|Texas Instruments Incorporated
| Marketing Part # : LMKDB1XXX
| Voltage Range : 1.8-3.3V
| Package-type: QFN
| #pins/pkg drawing : 40-pin RSL
[IBIS Ver] 3.2
[File name] lmkdb1xxx.ibs
[File Rev] 1.0
[Date] 09/07/2023
[Source]
| Texas Instruments Incorporated.
| 12500 TI Blvd
| Dallas, TX -75243
[Notes] Revision History:
| Rev 1.0: 09/07/2023
| - Initial version of the model
| - Model generated from simulations in TISPICE/SPECTRE
| - C_comp although listed in numerical order of value are
| obtained from varying PVT conditions. For PVT conditions for
| each specific value refer the buffer description under
| respective [Model]. IBIS model user is responsible for using
| appropriate C_comp to simulate for Signal Integrity.
| - Warnings regarding combined Non-monotonicity of various models have been
| reviewed and considered minor and can be ignored.
[Disclaimer]
| This model is designed as an aid for customers of Texas Instruments.
| TI and its licensors and suppliers make no warranties, either expressed
| or implied, with respect to this model, including the warranties of
| merchantability or fitness for a particular purpose. The model is
| provided solely on an "as is" basis. The entire risk as to its quality
| and performance is with the customer.
| This model is subject to change without notice. Texas Instruments
| Incorporated is not responsible for updating this model.
[Copyright]
(C) Copyright 2023 Texas Instruments Incorporated. All rights reserved.
| Component LMKDB1120 (per package)
[Component] LMKDB1120
[Manufacturer] Texas Instruments Incorporated
[Package] |80 GQFN
| variable typ min max
R_pkg 0.111 0.052 0.169
L_pkg 2.02nH 1.12nH 2.9nH
C_pkg 0.163pF 0.062pF 0.264pF
| pin number (pin name) mapping to model name
[Pin] signal_name model_name R_pin L_pin C_pin
1   CLKIN_P   ck_in   NA   NA   NA
2   CLKIN_N   ck_in   NA   NA   NA
3   CLK0_P   ck_out   NA   NA   NA
4   CLK0_N   ck_out   NA   NA   NA
5   CLK1_P   ck_out   NA   NA   NA
6   CLK1_N   ck_out   NA   NA   NA
7   CLK2_P   ck_out   NA   NA   NA
8   CLK2_N   ck_out   NA   NA   NA
9   CLK3_P   ck_out   NA   NA   NA
10   CLK3_N   ck_out   NA   NA   NA
11   CLK4_P   ck_out   NA   NA   NA
12   CLK4_N   ck_out   NA   NA   NA
13   CLK5_P   ck_out   NA   NA   NA
14   CLK5_N   ck_out   NA   NA   NA
15   CLK6_P   ck_out   NA   NA   NA
16   CLK6_N   ck_out   NA   NA   NA
17   CLK7_P   ck_out   NA   NA   NA
18   CLK7_N   ck_out   NA   NA   NA
19   CLK8_P   ck_out   NA   NA   NA
20   CLK8_N   ck_out   NA   NA   NA
21   CLK9_P   ck_out   NA   NA   NA
22   CLK9_N   ck_out   NA   NA   NA
23   CLK10_P   ck_out   NA   NA   NA
24   CLK10_N   ck_out   NA   NA   NA
25   CLK11_P   ck_out   NA   NA   NA
26   CLK11_N   ck_out   NA   NA   NA
27   CLK12_P   ck_out   NA   NA   NA
28   CLK12_N   ck_out   NA   NA   NA
29   CLK13_P   ck_out   NA   NA   NA
30   CLK13_N   ck_out   NA   NA   NA
31   CLK14_P   ck_out   NA   NA   NA
32   CLK14_N   ck_out   NA   NA   NA
33   CLK15_P   ck_out   NA   NA   NA
34   CLK15_N   ck_out   NA   NA   NA
35   CLK16_P   ck_out   NA   NA   NA
36   CLK16_N   ck_out   NA   NA   NA
37   CLK17_P   ck_out   NA   NA   NA
38   CLK17_N   ck_out   NA   NA   NA
39   CLK18_P   ck_out   NA   NA   NA
40   CLK18_N   ck_out   NA   NA   NA
41   CLK19_P   ck_out   NA   NA   NA
42   CLK19_N   ck_out   NA   NA   NA
43   POWERGD_POWERDNb   gpi   NA   NA   NA
44   OE5B/SBI_IN   gpi   NA   NA   NA
45   OE6B/SBI_CLK   gpi   NA   NA   NA
46   OE7B   gpi   NA   NA   NA
47   OE8B   gpi   NA   NA   NA
48   OE9B   gpi   NA   NA   NA
49   OE10B/SHIFT_LDb   gpi   NA   NA   NA
50   OE11B   gpi   NA   NA   NA
51   OE12B   gpi   NA   NA   NA
52   SADR0   strap_in   NA   NA   NA
53   SADR1   strap_in   NA   NA   NA
54   VDD   POWER   NA   NA   NA
55   SBEN   gpi   NA   NA   NA
56   VDDR   POWER   NA   NA   NA
57   SMB_DATA   smbdat   NA   NA   NA
58   SMB_CLK   smbclk   NA   NA   NA
59   SBI_OUT   nc   NA   NA   NA
60   OE0B   gpi   NA   NA   NA
61   OE1B   gpi   NA   NA   NA
62   OE2B   gpi   NA   NA   NA
63   OE3B   gpi   NA   NA   NA
64   OE4B   gpi   NA   NA   NA
65   OE13B   gpi   NA   NA   NA
66   OE14B   gpi   NA   NA   NA
67   OE15B   gpi   NA   NA   NA
68   OE16B   gpi   NA   NA   NA
69   OE17B   gpi   NA   NA   NA
70   OE18B   gpi   NA   NA   NA
71   OE19B   gpi   NA   NA   NA
72   LOSB   los   NA   NA   NA
[Diff Pin]   inv_pin   vdiff   tdelay_typ  tdelay_min  tdelay_max
1   2   10m   NA   NA   NA
3   4   NA   NA   NA   NA
5   6   NA   NA   NA   NA
7   8   NA   NA   NA   NA
9   10   NA   NA   NA   NA
11   12   NA   NA   NA   NA
13   14   NA   NA   NA   NA
15   16   NA   NA   NA   NA
17   18   NA   NA   NA   NA
19   20   NA   NA   NA   NA
21   22   NA   NA   NA   NA
23   24   NA   NA   NA   NA
25   26   NA   NA   NA   NA
27   28   NA   NA   NA   NA
29   30   NA   NA   NA   NA
31   32   NA   NA   NA   NA
33   34   NA   NA   NA   NA
35   36   NA   NA   NA   NA
37   38   NA   NA   NA   NA
39   40   NA   NA   NA   NA
41   42   NA   NA   NA   NA
| Component LMKDB1108 (per package)
[Component] LMKDB1108
[Manufacturer] Texas Instruments Incorporated
[Package] |40 QFN
| variable typ min max
R_pkg 0.111 0.052 0.169
L_pkg 2.02nH 1.12nH 2.9nH
C_pkg 0.163pF 0.062pF 0.264pF
| pin number (pin name) mapping to model name
[Pin] signal_name model_name R_pin L_pin C_pin
1   LOSb   los   NA   NA   NA
2   SLEWRATE_SEL   gpi   NA   NA   NA
3   SADR0_TRI   strap_in   NA   NA   NA
4   SADR1_TRI   strap_in   NA   NA   NA
5   SMB_DATA   smbdat   NA   NA   NA
6   SMB_CLK   smbclk   NA   NA   NA
7   VDDR   POWER   NA   NA   NA
8   CLKIN_P   ck_in   NA   NA   NA
9   CLKIN_N   ck_in   NA   NA   NA
10   VDD   POWER   NA   NA   NA
11   SBI_EN   gpi   NA   NA   NA
12   POWERGD_POWERDNb   gpi   NA   NA   NA
13   VDD   POWER   NA   NA   NA
14   OE0B/SHFT_LDb   gpi   NA   NA   NA
15   CLK0_P   ck_out   NA   NA   NA
16   CLK0_N   ck_out   NA   NA   NA
17   CLK1_P   ck_out   NA   NA   NA
18   CLK1_N   ck_out   NA   NA   NA
19   OE1B/SBI_IN   gpi   NA   NA   NA
20   VDD   POWER   NA   NA   NA
21   OE2B   gpi   NA   NA   NA
22   CLK2_P   ck_out   NA   NA   NA
23   CLK2_N   ck_out   NA   NA   NA
24   CLK3_P   ck_out   NA   NA   NA
25   CLK3_N   ck_out   NA   NA   NA
26   VDD   POWER   NA   NA   NA
27   OE3B   gpi   NA   NA   NA
28   CLK4_P   ck_out   NA   NA   NA
29   CLK4_N   ck_out   NA   NA   NA
30   OE4B/SBI_CLK   gpi   NA   NA   NA
31   CLK5_P   ck_out   NA   NA   NA
32   CLK5_N   ck_out   NA   NA   NA
33   OE5B   gpi   NA   NA   NA
34   OE6B/SBI_OUT   gpi   NA   NA   NA
35   CLK6_P   ck_out   NA   NA   NA
36   CLK6_N   ck_out   NA   NA   NA
37   VDD   POWER   NA   NA   NA
38   CLK7_P   ck_out   NA   NA   NA
39   CLK7_N   ck_out   NA   NA   NA
40   OE7B   gpi   NA   NA   NA
[Diff Pin]   inv_pin   vdiff   tdelay_typ  tdelay_min  tdelay_max
8   9   10m   NA   NA   NA
15   16   NA   NA   NA   NA
17   18   NA   NA   NA   NA
22   23   NA   NA   NA   NA
24   25   NA   NA   NA   NA
28   29   NA   NA   NA   NA
31   32   NA   NA   NA   NA
35   36   NA   NA   NA   NA
38   39   NA   NA   NA   NA
| Component LMKDB1104 (per package)
[Component] LMKDB1104
[Manufacturer] Texas Instruments Incorporated
[Package] |28 QFN
| variable typ min max
R_pkg 0.111 0.052 0.169
L_pkg 2.02nH 1.12nH 2.9nH
C_pkg 0.163pF 0.062pF 0.264pF
| pin number (pin name) mapping to model name
[Pin] signal_name model_name R_pin L_pin C_pin
1   SADR0_TRI   strap_in   NA   NA   NA
2   SADR1_TRI   strap_in   NA   NA   NA
3   SMB_DATA   smbdat   NA   NA   NA
4   SMB_CLK   smbclk   NA   NA   NA
5   VDDR   POWER   NA   NA   NA
6   CLKIN_P   ck_in   NA   NA   NA
7   CLKIN_N   ck_in   NA   NA   NA
8   SBI_EN   gpi   NA   NA   NA
9   POWERGD_POWERDNb   gpi   NA   NA   NA
10   VDD   POWER   NA   NA   NA
11   OE0B/SHFT_LDb   gpi   NA   NA   NA
12   CLK0_P   ck_out   NA   NA   NA
13   CLK0_N   ck_out   NA   NA   NA
14   OE1B/SBI_IN   gpi   NA   NA   NA
15   VDD   POWER   NA   NA   NA
16   CLK1_P   ck_out   NA   NA   NA
17   CLK1_N   ck_out   NA   NA   NA
18   VDD   POWER   NA   NA   NA
19   CLK2_P   ck_out   NA   NA   NA
20   CLK2_N   ck_out   NA   NA   NA
21   OE2B/SBI_CLK   gpi   NA   NA   NA
22   OE3B/SBI_OUT   gpi   NA   NA   NA
23   CLK3_P   ck_out   NA   NA   NA
24   CLK3_N   ck_out   NA   NA   NA
25   VDD   POWER   NA   NA   NA
27   SLEWRATE_SEL   gpi   NA   NA   NA
28   LOSb   los   NA   NA   NA
[Diff Pin]   inv_pin   vdiff   tdelay_typ  tdelay_min  tdelay_max
6   7   10m   NA   NA   NA
12   13   NA   NA   NA   NA
16   17   NA   NA   NA   NA
19   20   NA   NA   NA   NA
23   24   NA   NA   NA   NA
| Component LMKDB1102 (per package)
[Component] LMKDB1102
[Manufacturer] Texas Instruments Incorporated
[Package] |20 QFN
| variable typ min max
R_pkg 0.111 0.052 0.169
L_pkg 2.02nH 1.12nH 2.9nH
C_pkg 0.163pF 0.062pF 0.264pF
| pin number (pin name) mapping to model name
[Pin] signal_name model_name R_pin L_pin C_pin
1   CLKIN_P   ck_in   NA   NA   NA
2   CLKIN_N   ck_in   NA   NA   NA
3   VDD_IN   POWER   NA   NA   NA
6   VDD_IN   POWER   NA   NA   NA
7   GND   GND   NA   NA   NA
8   VDDO   POWER   NA   NA   NA
9   CLK2_P   ck_out   NA   NA   NA
10   CLK2_N   ck_out   NA   NA   NA
11   ZOUTSEL   gpi   NA   NA   NA
12   OE2B   gpi   NA   NA   NA
13   LOSb   los   NA   NA   NA
14   VDD   POWER   NA   NA   NA
15   OE1B   gpi   NA   NA   NA
16   CLK1_P   ck_out   NA   NA   NA
17   CLK1_N   ck_out   NA   NA   NA
18   VDDO   POWER   NA   NA   NA
19   VDD_DIG   POWER   NA   NA   NA
20   GND   GND   NA   NA   NA
[Diff Pin]   inv_pin   vdiff   tdelay_typ  tdelay_min  tdelay_max
1   2   10m   NA   NA   NA
9   10   NA   NA   NA   NA
16   17   NA   NA   NA   NA
| Component LMKDB1204 (per package)
[Component] LMKDB1204
[Manufacturer] Texas Instruments Incorporated
[Package] |28 QFN
| variable typ min max
R_pkg 0.111 0.052 0.169
L_pkg 2.02nH 1.12nH 2.9nH
C_pkg 0.163pF 0.062pF 0.264pF
| pin number (pin name) mapping to model name
[Pin] signal_name model_name R_pin L_pin C_pin
1   POWERGD_POWERDNb   gpi   NA   NA   NA
2   CLKIN0_P   ck_in   NA   NA   NA
3   CLKIN0_N   ck_in   NA   NA   NA
4   VDD_IN0   POWER   NA   NA   NA
5   CLKIN1_P   ck_in   NA   NA   NA
6   CLKIN1_N   ck_in   NA   NA   NA
7   VDD_IN1   POWER   NA   NA   NA
8   CLKSEL_TRI   strap_in   NA   NA   NA
9   OE3B   gpi   NA   NA   NA
10   CLK3_P   ck_out   NA   NA   NA
11   CLK3_N   ck_out   NA   NA   NA
12   VDD_BANK1   POWER   NA   NA   NA
13   CLK2_P   ck_out   NA   NA   NA
14   CLK2_N   ck_out   NA   NA   NA
16   OE2B   gpi   NA   NA   NA
17   LOSb   los   NA   NA   NA
18   VDD   POWER   NA   NA   NA
19   OE1B   gpi   NA   NA   NA
20   CLK1_P   ck_out   NA   NA   NA
21   CLK1_N   ck_out   NA   NA   NA
22   VDD_BANK0   POWER   NA   NA   NA
23   CLK0_P   ck_out   NA   NA   NA
24   CLK0_N   ck_out   NA   NA   NA
25   OE0B   gpi   NA   NA   NA
26   VDD_DIG   POWER   NA   NA   NA
27   GND   GND   NA   NA   NA
28   ZOUTSEL   gpi   NA   NA   NA
[Diff Pin]   inv_pin   vdiff   tdelay_typ  tdelay_min  tdelay_max
2   3   10m   NA   NA   NA
5   6   10m   NA   NA   NA
10   11   NA   NA   NA   NA
13   14   NA   NA   NA   NA
20   21   NA   NA   NA   NA
23   24   NA   NA   NA   NA
| Component LMKDB1202 (per package)
[Component] LMKDB1202
[Manufacturer] Texas Instruments Incorporated
[Package] |20 QFN
| variable typ min max
R_pkg 0.111 0.052 0.169
L_pkg 2.02nH 1.12nH 2.9nH
C_pkg 0.163pF 0.062pF 0.264pF
| pin number (pin name) mapping to model name
[Pin] signal_name model_name R_pin L_pin C_pin
1   CLKIN0_P   ck_in   NA   NA   NA
2   CLKIN0_N   ck_in   NA   NA   NA
3   VDD_IN0   POWER   NA   NA   NA
4   CLKIN1_P   ck_in   NA   NA   NA
5   CLKIN1_N   ck_in   NA   NA   NA
6   VDD_IN1   POWER   NA   NA   NA
7   CLKSEL_TRI   strap_in   NA   NA   NA
8   VDD_BANK1   POWER   NA   NA   NA
9   CLK2_P   ck_out   NA   NA   NA
10   CLK2_N   ck_out   NA   NA   NA
11   ZOUTSEL   gpi   NA   NA   NA
12   OE2B   gpi   NA   NA   NA
13   LOSb   los   NA   NA   NA
14   VDD   POWER   NA   NA   NA
15   OE1B   gpi   NA   NA   NA
16   CLK1_P   ck_out   NA   NA   NA
17   CLK1_N   ck_out   NA   NA   NA
18   VDD_BANK0   POWER   NA   NA   NA
19   VDD_DIG   POWER   NA   NA   NA
20   GND   GND   NA   NA   NA
[Diff Pin]   inv_pin   vdiff   tdelay_typ  tdelay_min  tdelay_max
1   2   10m   NA   NA   NA
4   5   10m   NA   NA   NA
9   10   NA   NA   NA   NA
16   17   NA   NA   NA   NA
|***** end of component definition
| Model Selectors
|***Modify the following as it applies to a speciic model with multiple ****
|*** powver supply options or driver programmability *********
[Model Selector] ck_out
output_85 85ohm differential driver
output_100 100ohm differential driver
| Models and submodels in the file (8): ck_in (Input), gpi (Input), output_85 (Output), output_100 (Output), smbclk (Input), smbdat (I/O_open_drain), strap_in (Input), los (Open_drain)
